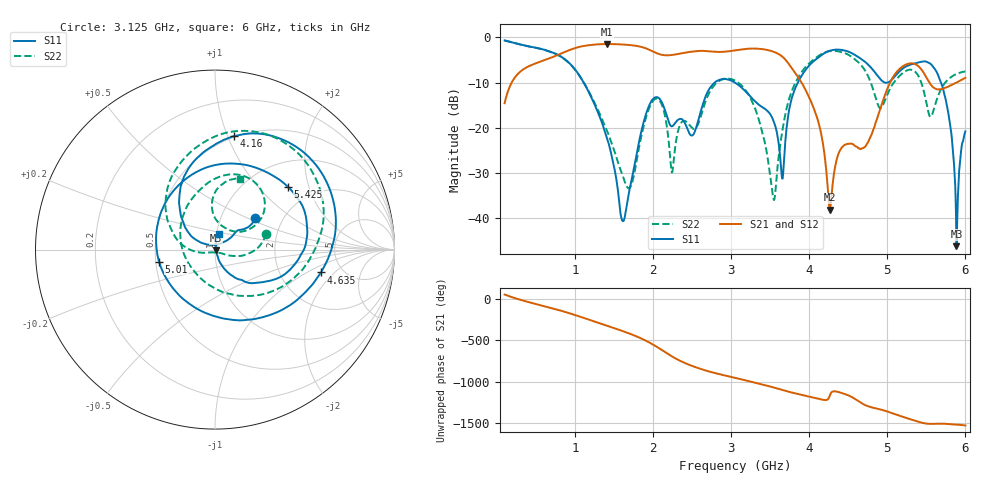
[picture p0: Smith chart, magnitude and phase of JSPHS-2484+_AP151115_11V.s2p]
!Mini-Circuits Laboratory
!S-Parameters
!Run/Lot/Date Code:MF33450/NA/1551
!Fixture/SN/Due: 90-4-20-21/70546/03/17/16
!Connection:PORT<IN> - pin<1>; PORT<OUT> - pin<7>;PORT<BIAS> - pin<4>;
!Tested With:PORT EXTENTION
!Network Analyzer:AG E5071C/74883/05/12/16
!Created: 01-07-2016 at 14:10:48
!MODEL: JSPHS-2484+
!S/N: V=11V
# MHZ S DB R 50
!Frequency  S11 dB  S11 DEG  S21 dB  S21 DEG  S12 dB  S12 DEG  S22 dB  S22 DEG
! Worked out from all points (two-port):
!   1181 points, 100 MHz to 6 GHz, reference 50 ohm
!   highest |S21| = -1.45 dB at 1.41 GHz (marker M1); lowest = -38.1 dB at 4.265 GHz (marker M2)
!   |S21| within 3 dB of the highest: 700.4 MHz to 3.67 GHz (2.97 GHz wide, 136 % of centre)
!   lowest |S11| = -46.1 dB at 5.885 GHz (marker M3), VSWR 1.01, Z = 50.4 - j0.294 ohm
!   |S11| at or under -10 dB: 1.114 GHz to 2.787 GHz (1.674 GHz wide, 85.8 % of centre); 3.051 GHz to 3.855 GHz (804.4 MHz wide, 23.3 % of centre); 5.688 GHz to end of sweep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
!   |S22| runs from -35.9 to -0.7 dB; largest |S21 - S12| = 0.0024
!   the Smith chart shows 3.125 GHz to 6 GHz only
!   S11 on the Smith chart (normalised r, x): 3.125 GHz: 1.45, +0.55; 4.16 GHz: 0.49, +1.06; 4.635 GHz: 3.45, -1.38; 5.01 GHz: 0.52, -0.08; 5.425 GHz: 1.50, +1.47; 6 GHz: 1.03, +0.18
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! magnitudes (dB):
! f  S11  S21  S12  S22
! 100 MHz  -0.7  -14.5  -14.5  -0.7
! 1.085 GHz  -9.2  -2.0  -2.0  -9.2
! 1.41 GHz  -22.2  -1.5  -1.4  -20.5
! 1.62 GHz  -40.6  -1.6  -1.6  -30.9
! 2.07 GHz  -13.3  -3.6  -3.6  -13.7
! 2.245 GHz  -19.6  -3.9  -3.9  -29.8
! 3.05 GHz  -10.0  -2.9  -2.9  -9.5
! 3.125 GHz  -10.9  -2.7  -2.7  -10.4
! 3.545 GHz  -18.5  -3.2  -3.2  -35.8
! 3.655 GHz  -31.2  -4.2  -4.2  -20.8
! 3.78 GHz  -13.2  -6.9  -6.8  -11.7
! 4.035 GHz  -5.6  -14.6  -14.6  -5.2
! 4.16 GHz  -3.9  -21.9  -21.9  -3.6
! 4.265 GHz  -2.9  -38.1  -38.2  -3.0
! 4.635 GHz  -4.4  -24.5  -24.7  -5.6
! 5.01 GHz  -9.9  -10.9  -10.9  -12.2
! 5.02 GHz  -9.8  -10.5  -10.5  -11.8
! 5.425 GHz  -5.4  -6.8  -6.8  -9.5
! 5.555 GHz  -5.8  -10.4  -10.4  -17.5
! 5.73 GHz  -12.6  -11.2  -11.2  -10.2
! 5.885 GHz  -46.1  -10.0  -10.0  -8.1
! 6 GHz  -20.8  -8.9  -8.9  -7.5
